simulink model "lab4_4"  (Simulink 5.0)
settings: Solver=FixedStepDiscrete  StartTime=0.0  StopTime=0.5  FixedStep=T  RelTol=1e-3
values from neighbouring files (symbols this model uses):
  l1 = VREF-delta    (= 3.75)    [lab4_4.m]
  l2 = -VREF    (= -5)    [lab4_4.m]
  T = 1/Fsamp    (= 0.0001)    [lab4_4.m]
libraries: simulink x1

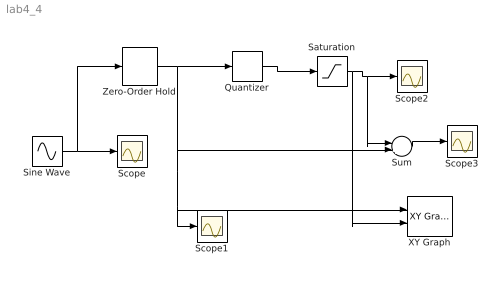
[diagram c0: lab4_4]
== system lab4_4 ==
  Quantizer : Quantizer  QuantizationInterval=delta
  Saturation : Saturate  UpperLimit=l1  LowerLimit=l2
  Scope{,1..3} (4 alike) : Scope
  Sine Wave : Sin  Amplitude=VREF-delta  Frequency=2*pi*10  SampleTime=0
  Sum : Sum  Inputs=|+-
  XY Graph : simulink/Sinks/XY Graph  xmin=-10  xmax=10  ymin=-10  ymax=10  st=T
  Zero-Order Hold : ZeroOrderHold  SampleTime=T
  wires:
  Sine Wave/1 -> Scope/1, Zero-Order Hold/1
  Zero-Order Hold/1 -> Quantizer/1, Sum/2, Scope1/1, XY Graph/1
  Quantizer/1 -> Saturation/1
  Saturation/1 -> Scope2/1, Sum/1, XY Graph/2
  Sum/1 -> Scope3/1
